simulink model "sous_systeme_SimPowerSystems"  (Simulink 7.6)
settings: Solver=ode3  StartTime=0.0  StopTime=0.02  RelTol=1e-3
InitFcn:
  | clc
  | clear all
  | close all
  | delete *.mat
StopFcn:
  | close all, clc
  | 
  | load UI_phaseA.mat
  | plotyy(x(1,:),x(2,:), x(1,:),x(3,:))
  | grid
  | title('Courant et tension phase A')
  | xlabel('temps')
  | %axis([0 N 100 300])
  | delete *.mat, clear all
libraries: powerlib x7

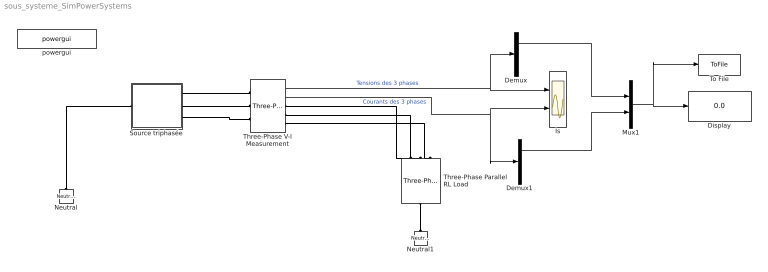
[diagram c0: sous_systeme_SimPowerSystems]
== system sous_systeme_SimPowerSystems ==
  Demux : Demux  Outputs=3
  Demux1 : Demux  Outputs=3
  Display : Display
  Is : Scope  NumInputPorts=2
  Mux1 : Mux  Inputs=2
  Neutral : powerlib/Elements/Neutral  DialogController=POWERSYS.PowerSysDialog  PhysicalDomain=powersysdomain  SubClassName=unknown  LeftPortType=p1  RightPortType=p1  LConnTagsString=a  NodeNumber=1
  Neutral1 : powerlib/Elements/Neutral  DialogController=POWERSYS.PowerSysDialog  PhysicalDomain=powersysdomain  SubClassName=unknown  LeftPortType=p1  RightPortType=p1  LConnTagsString=a  NodeNumber=1
  Source triphasée : Subsystem
  Three-Phase Parallel RL Load : powerlib/Elements/Three-Phase Parallel RLC Load  DialogController=POWERSYS.PowerSysDialog  PhysicalDomain=powersysdomain  SubClassName=unknown  LeftPortType=p1  RightPortType=p1  LConnTagsString=A|B|C  RConnTagsString=N  Configuration=Y (neutral)  NominalVoltage=230/sqrt(2)  NominalFrequency=60  ActivePower=1e3  InductivePower=10  CapacitivePower=0  Measurements=None
  Three-Phase V-I Measurement : powerlib/Measurements/Three-Phase V-I Measurement  DialogController=POWERSYS.PowerSysDialog  SystemSampleTime=-1  VoltageMeasurement=phase-to-phase  SetLabelV=off  LabelV=Vabc  Vpu=off  VpuLL=off  CurrentMeasurement=yes  SetLabelI=off  LabelI=Iabc  Ipu=off  Pbase=100e6  Vbase=500e3  OutputType=Complex  PhasorSimulation=off  PSBequivalent=0
  To File : ToFile  Filename=UI_phaseA  MatrixName=x
  powergui : powerlib/powergui  Priority=1  SystemSampleTime=-1  SimulationMode=Discrete  SampleTime=50e-6  frequency=60  SPID=off  DisableSnubberDevices=off  DisableRonSwitches=off  DisableVfSwitches=off  SwTol=0  Interpol=off  frequencyindice=60  echomessages=off  HookPort=off  DisplayEquations=off  FunctionMessages=off  EnableUseOfTLC=off  x0status=blocks  RestoreLinks=warning  ResistiveCurrentMeasurement=off  Frange=[0:2:200]  Ylog=off  Xlog=on  ShowGrid=on  save=off  variable=ZData  structure=ScopeData  ZoomFFT=off  StartTime=0.0  cycles=1  DisplayStyle=1  fundamental=60  FreqAxis=off  MaxFrequency=1000  frequencyindicesteady=1  display=off  methode=off
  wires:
  Three-Phase V-I Measurement/1 -> Is/1, Demux/1  "Tensions des 3 phases"
  Three-Phase V-I Measurement/2 -> Is/2, Demux1/1  "Courants des 3 phases"
  Demux1/1 -> Mux1/2
  Demux/1 -> Mux1/1
  Mux1/1 -> Display/1, To File/1
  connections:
  Three-Phase V-I Measurement/RConn3 -- Three-Phase Parallel RL Load/LConn3
  Three-Phase V-I Measurement/RConn2 -- Three-Phase Parallel RL Load/LConn2
  Three-Phase V-I Measurement/RConn1 -- Three-Phase Parallel RL Load/LConn1
  Neutral/LConn1 -- Source triphasée/LConn1
  Three-Phase Parallel RL Load/RConn1 -- Neutral1/LConn1
  Source triphasée/RConn1 -- Three-Phase V-I Measurement/LConn1
  Source triphasée/RConn2 -- Three-Phase V-I Measurement/LConn2
  Source triphasée/RConn3 -- Three-Phase V-I Measurement/LConn3

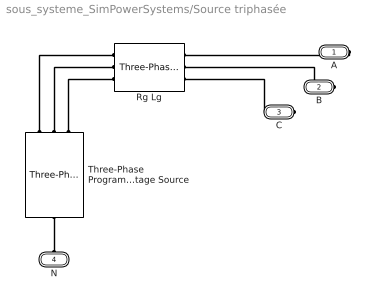
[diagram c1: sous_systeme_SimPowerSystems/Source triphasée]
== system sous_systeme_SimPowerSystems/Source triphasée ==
  Rg Lg : powerlib/Elements/Three-Phase Parallel RLC Branch  DialogController=POWERSYS.PowerSysDialog  PhysicalDomain=powersysdomain  SubClassName=unknown  LeftPortType=p1  RightPortType=p1  LConnTagsString=A|B|C  RConnTagsString=A|B|C  BranchType=RL  Resistance=1  Inductance=1e-3  Capacitance=1e-6  Measurements=None
  Three-Phase Programmable Voltage Source : powerlib/Electrical Sources/Three-Phase Programmable Voltage Source  DialogController=POWERSYS.PowerSysDialog  SystemSampleTime=-1  PositiveSequence="[220e6/sqrt(2)  0 60]"  VariationEntity=None  VariationType=Step  VariationStep=0.5  VariationRate=10  VariationMagnitude=0.3  VariationFrequency=2  VariationTiming=[1 2]  VariationPhaseA=off  Amplitudes=[1 0.8 1.2 1.0]  TimeValues=[0 0.1 0.15 0.2]  HarmonicGeneration=off  HarmonicA=[3 0.2 -25 0]  HarmonicB=[2 0.15 35 2]  Timing="[0.05  3]"
  A : PMIOPort  Port=1  Side=Right
  B : PMIOPort  Port=2  Side=Right
  C : PMIOPort  Port=3  Side=Right
  N : PMIOPort  Port=4  Side=Left
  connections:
  Three-Phase Programmable Voltage Source/RConn1 -- Rg Lg/LConn1
  Three-Phase Programmable Voltage Source/RConn2 -- Rg Lg/LConn2
  Three-Phase Programmable Voltage Source/RConn3 -- Rg Lg/LConn3
  A/RConn1 -- Rg Lg/RConn1
  B/RConn1 -- Rg Lg/RConn2
  C/RConn1 -- Rg Lg/RConn3
  N/RConn1 -- Three-Phase Programmable Voltage Source/LConn1
